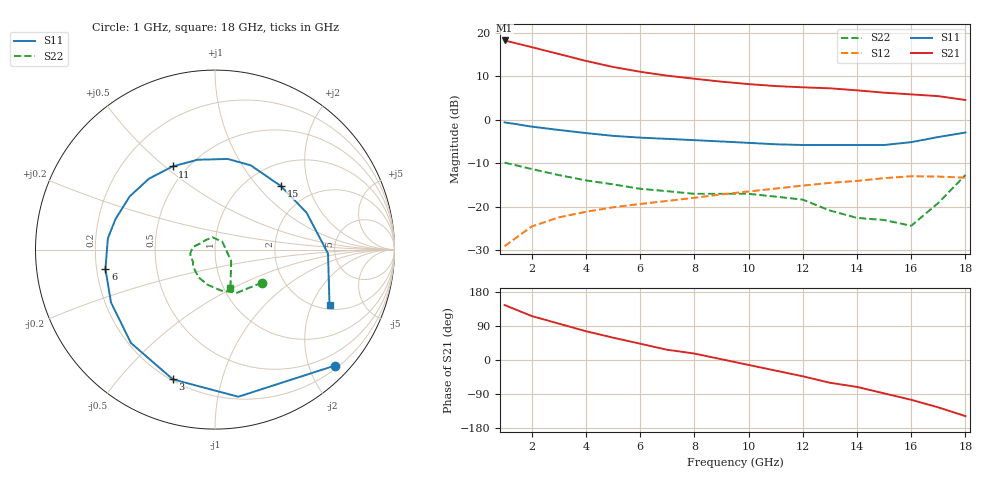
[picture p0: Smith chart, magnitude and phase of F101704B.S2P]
!!ATF-10170
!S-PARAMETERS at Vds=4V  Id=70mA.  LAST UPDATED 07-22-92
# ghz s ma r 50
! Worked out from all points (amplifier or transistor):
!   18 points, 1 GHz to 18 GHz, reference 50 ohm
!   highest |S21| = 18.2 dB at 1 GHz (marker M1)
!   |S21| within 3 dB of that: start of sweep to 2.927 GHz
!   unconditionally stable (mu >= 1): 8.858 GHz to 16.78 GHz
!   at 4 GHz: K = 0.67, MSG = 17.4 dB, |S12| = -21.2 dB
!   at 10 GHz: K = 1.03, MAG = 11.4 dB, |S12| = -16.5 dB
!   at 18 GHz: K = 0.99, MSG = 8.9 dB, |S12| = -13.4 dB
!   S11 on the Smith chart (normalised r, x): 1 GHz: 0.26, -2.45; 3 GHz: 0.21, -0.71; 6 GHz: 0.24, -0.08; 11 GHz: 0.42, +0.53; 15 GHz: 1.41, +1.35; 18 GHz: 2.18, -2.73
1  0.93 -44.0  8.13 145.0  0.035 64.0  0.32 -35.0
2  0.83 -81.0  6.81 116.0  0.059 47.0  0.27 -63.0
3  0.76 -108.0  5.68 96.0  0.075 38.0  0.23 -82.0
4  0.7 -132.0  4.73 76.0  0.087 27.0  0.2 -102.0
5  0.65 -153.0  4.03 59.0  0.098 18.0  0.18 -120.0
6  0.62 -170.0  3.55 43.0  0.107 10.0  0.16 -135.0
7  0.6 174.0  3.2 27.0  0.116 2.0  0.15 -145.0
8  0.58 163.0  2.95 17.0  0.126 -2.0  0.14 -151.0
9  0.56 148.0  2.73 2.0  0.138 -11.0  0.14 -161.0
10  0.54 133.0  2.56 -13.0  0.149 -21.0  0.14 -171.0
11  0.52 117.0  2.43 -28.0  0.161 -31.0  0.13 -179.0
12  0.51 101.0  2.35 -43.0  0.174 -43.0  0.12 172.0
13  0.51 82.0  2.29 -60.0  0.187 -55.0  0.09 158.0
14  0.51 67.0  2.17 -71.0  0.197 -62.0  0.074 134.0
15  0.51 44.0  2.04 -88.0  0.212 -76.0  0.07 102.0
16  0.55 22.0  1.95 -105.0  0.223 -93.0  0.06 48.0
17  0.63 -2.0  1.86 -125.0  0.221 -111.0  0.11 -35.0
18  0.71 -26.0  1.68 -148.0  0.215 -127.0  0.23 -68.0
